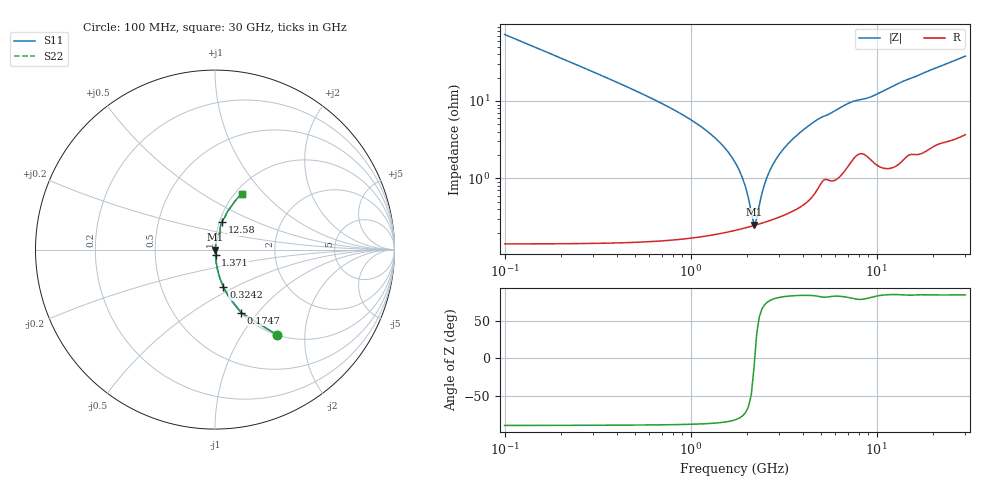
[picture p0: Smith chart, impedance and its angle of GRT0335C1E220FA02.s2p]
!Murata Part Number: GRT0335C1E220FA02
!These Parameters are Measured in Series Mode Connection
!Data Generated on Jun 19, 2026
!  o--ll--o
!Port1  Port2
!  o------o
!Operation Temp=25[degC], DC Bias Voltage=0[V]
!Freq. Start=100[MHz] Stop=30[GHz] 401[Steps]
# Hz S RI R 50
!Freq.(Hz) S11(Real) S11(Imag) S21(Real) S21(Imag) S12(Real) S12(Imag) S22(Real) S22(Imag)
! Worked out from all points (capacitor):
!   401 points, 100 MHz to 30 GHz, reference 50 ohm
!   read as one part in series: C = 22 pF near 249.5 MHz
!   lowest |Z| = 252 mohm at 2.193 GHz (marker M1)
!   series resonance near 2.211 GHz, so ESL is about 240 pH
!   S11 on the Smith chart (normalised r, x): 100 MHz: 1.00, -1.44; 174.8 MHz: 1.00, -0.82; 324.2 MHz: 1.00, -0.44; 1.371 GHz: 1.00, -0.06; 12.58 GHz: 1.03, +0.32; 30 GHz: 1.07, +0.76
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1e8  0.3429 -0.4737  0.6571 0.4737  0.6571 0.4737  0.3429 -0.4737
1.7475e8  0.1456 -0.351  0.8544 0.351  0.8544 0.351  0.1456 -0.351
3.2425e8  0.0467 -0.2078  0.9533 0.2078  0.9533 0.2078  0.0467 -0.2078
6.2325e8  0.0128 -0.1052  0.9872 0.1052  0.9872 0.1052  0.0128 -0.1052
1.37075e9  0.00294 -0.0322  0.9971 0.0322  0.9971 0.0322  0.00294 -0.0322
1.7445e9  0.00238 -0.0155  0.9976 0.0155  0.9976 0.0155  0.00238 -0.0155
1.894e9  0.00234 -0.0101  0.9977 0.0101  0.9977 0.0101  0.00234 -0.0101
2.11825e9  0.00241 -0.00277  0.9976 0.00277  0.9976 0.00277  0.00241 -0.00277
2.193e9  0.00246 -0.000518  0.9975 0.000518  0.9975 0.000518  0.00246 -0.000518
2.3425e9  0.00259 0.00376  0.9974 -0.00376  0.9974 -0.00376  0.00259 0.00376
2.56675e9  0.00286 0.00972  0.9971 -0.00972  0.9971 -0.00972  0.00286 0.00972
2.71625e9  0.00308 0.0135  0.9969 -0.0135  0.9969 -0.0135  0.00308 0.0135
3.16475e9  0.00389 0.0238  0.9961 -0.0238  0.9961 -0.0238  0.00389 0.0238
3.987e9  0.0061 0.0407  0.9939 -0.0407  0.9939 -0.0407  0.0061 0.0407
5.10825e9  0.0127 0.0603  0.9873 -0.0603  0.9873 -0.0603  0.0127 0.0603
7.20125e9  0.0238 0.0904  0.9762 -0.0904  0.9762 -0.0904  0.0238 0.0904
1.01165e10  0.0287 0.1176  0.9713 -0.1176  0.9713 -0.1176  0.0287 0.1176
1.258325e10  0.038 0.1519  0.962 -0.1519  0.962 -0.1519  0.038 0.1519
1.505e10  0.0535 0.1786  0.9465 -0.1786  0.9465 -0.1786  0.0535 0.1786
2.005825e10  0.0823 0.2296  0.9177 -0.2296  0.9177 -0.2296  0.0823 0.2296
2.50665e10  0.1135 0.2723  0.8865 -0.2723  0.8865 -0.2723  0.1135 0.2723
3e10  0.1484 0.3102  0.8516 -0.3102  0.8516 -0.3102  0.1484 0.3102
